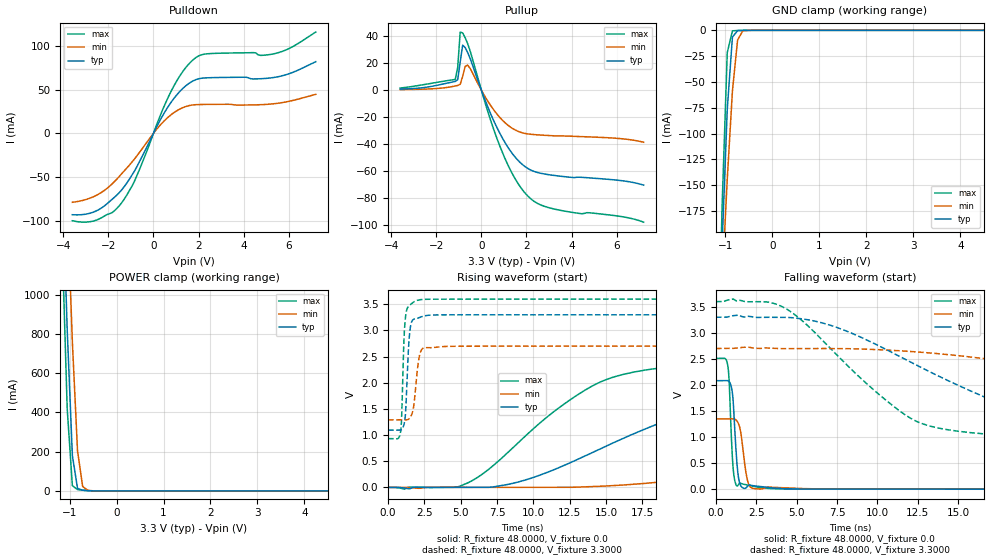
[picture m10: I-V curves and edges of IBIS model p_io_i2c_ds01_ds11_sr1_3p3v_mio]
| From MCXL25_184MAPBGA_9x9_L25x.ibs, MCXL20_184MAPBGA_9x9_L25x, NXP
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[Model] p_io_i2c_ds01_ds11_sr1_3p3v_mio
|   Model p_io_i2c_ds01_ds11_sr1_3p3v_mio
| This model was characterised for following simulation conditions:
| External (pad) voltage:
|   - Typ: 3.3V,   - Min: 2.7V,   - Max: 3.6V
| Library cells for typ/min/max conditions are connected as defined below:
|  pad - External Pad
|  ipp_do_lv - Core Input
|  ipp_obe_lv - Output Buffer Enable
|  IOGC - NC
|  REFH3V3 - REFH3V3
|  REFL3V3 - REFL3V3
|  ZI - NC
|  abut_ncal_vddio[1] - vddio
|  abut_ncal_vddio[2] - vddio
|  abut_ncal_vddio[3] - vssio
|  abut_ncal_vddio[4] - vddio
|  abut_ncal_vddio[5] - vddio
|  abut_ncal_vddio[6] - vssio
|  abut_pcal_vddio[1] - vssio
|  abut_pcal_vddio[2] - vssio
|  abut_pcal_vddio[3] - vddio
|  abut_pcal_vddio[4] - vssio
|  abut_pcal_vddio[5] - vssio
|  abut_pcal_vddio[6] - vddio
|  ipp_do_1p8v - ipp_do_1p8v
|  ipp_dse_lv[0] - vdd_lv
|  ipp_dse_lv[1] - vdd_lv
|  ipp_eftd_lv - NC
|  ipp_ina_mux_vddio - NC
|  ipp_ina_mux_vddio[0] - NC
|  ipp_ina_mux_vddio[1] - NC
|  ipp_ina_r0_vddio - NC
|  ipp_ina_r0a_vddio - NC
|  ipp_ina_r0b_vddio - NC
|  ipp_ina_r0c_vddio - NC
|  ipp_ina_r0d_vddio - NC
|  ipp_ina_r0e_vddio - NC
|  ipp_ina_r0f_vddio - NC
|  ipp_ina_r300_vddio - NC
|  ipp_ina_r300a_vddio - NC
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Model_type I/O
Polarity   Non-Inverting
Enable   Active-High
Vinl =   0.9900V
Vinh =   2.3100V
Vmeas =  1.6500V
Cref =   30.0000pF
Rref =   1.0000M
Vref =   3.3000V
C_comp   1.4149pF   1.3702pF   1.4746pF
|C_comp_pullup   0.5855pF   0.6309pF   0.5569pF
|C_comp_pulldown   0.7315pF   0.7413pF   0.7170pF
[Model Spec]
| variable   typ   min   max
Vinh   2.3100V   1.8900V   2.5200V
Vinl   0.9900V   0.8100V   1.0800V
[Temperature Range]   25.0000   0.1250k   -40.0000
[Voltage Range]   3.3000V   2.7000V   3.6000V
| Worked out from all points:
|   slope of the pulldown table from 0 to 0.495 V, typ, clamps not added: 20.5 ohm
|   slope of the pullup table from 0 to 0.495 V, typ, clamps not added: 23.9 ohm
|   GND clamp passes 1 mA (typ) near -0.75 V on its own axis
|   POWER clamp passes 1 mA (typ) near -0.57 V on its own axis
|   rising waveform, R_fixture 48.0000, V_fixture 0.0: 20-80 % time 11.6ns typ, 24.8ns min, 6.96ns max; typ from 0 V to 2.08 V
|   rising waveform, R_fixture 48.0000, V_fixture 3.3000: 20-80 % time 229ps typ, 322ps min, 191ps max; typ from 1.09 V to 3.3 V
|   falling waveform, R_fixture 48.0000, V_fixture 0.0: 20-80 % time 251ps typ, 343ps min, 212ps max; typ from 2.08 V to 0 V
|   falling waveform, R_fixture 48.0000, V_fixture 3.3000: 20-80 % time 9.25ns typ, 20.1ns min, 5.61ns max; typ from 3.3 V to 1.09 V
[Pulldown]
|Voltage   I(typ)   I(min)   I(max)
-3.6V     -93.31mA   -79.05mA   -100.2mA
-2.5V     -88.48mA   -70.63mA   -99.19mA
-1.84V    -75.78mA   -58.1mA    -91mA
-1.4V     -64.51mA   -45.95mA   -79.27mA
-850mV    -43.59mA   -29.61mA   -55.29mA
140mV     7.403mA    4.641mA    9.826mA
800mV     36.32mA    21.74mA    49.15mA
1.35V     52.7mA     30.01mA    72.7mA
1.79V     60.61mA    32.73mA    85.13mA
2.45V     63.81mA    33.25mA    91.42mA
5.42V     64.46mA    34.22mA    91.77mA
7.2V      82.23mA    44.78mA    116.2mA
[Pullup]
|Voltage   I(typ)   I(min)   I(max)
-3.6V     785.4uA    423.2uA    1.608mA
-1.16V    6.455mA    3.098mA    7.926mA
-1.05V    7.777mA    3.482mA    16.99mA
-940mV    20.9mA     4.372mA    43.05mA
-830mV    33.33mA    10.25mA    42.41mA
-720mV    31.61mA    17.65mA    38.91mA
-610mV    27.98mA    18.58mA    34.56mA
820mV     -32.01mA   -20.24mA   -41.48mA
1.48V     -49.28mA   -29.34mA   -65.19mA
2.03V     -57.72mA   -32.35mA   -77.98mA
3.24V     -63.24mA   -33.85mA   -88.14mA
7.2V      -70.41mA   -38.61mA   -97.87mA
[GND_clamp]
|Voltage   I(typ)   I(min)   I(max)
-3.6V     -4.327A    -3.181A    -5.901A
-1.18V    -358.9mA   -350.6mA   -379.3mA
-1.07V    -208.2mA   -244.2mA   -170.8mA
-960mV    -76.59mA   -144.3mA   -21.58mA
-850mV    -6.561mA   -58.74mA   -511.4uA
-740mV    -273.3uA   -9.382mA   -185.3uA
-630mV    -73.8uA    -593.1uA   -77.52uA
-410mV    -3.432uA   -9.016uA   -2.104uA
7.2V      0A         0A         0A
[POWER_clamp]
|Voltage   I(typ)   I(min)   I(max)
-3.6V     20.44A     18.76A     22.48A
-1.16V    1.647A     2.216A     1.289A
-1.05V    823.6mA    1.482A     419.2mA
-940mV    180.4mA    758.9mA    26.72mA
-830mV    12.56mA    202.9mA    6.794mA
-720mV    3.422mA    22.23mA    3.58mA
-610mV    1.373mA    2.923mA    1.344mA
7.2V      0A         0A         0A
[Ramp]
| variable   typ   min   max
dV/dt_r  1.2488/11.6455n   0.8046/24.8064n   1.5056/6.9631n
dV/dt_f  1.3236/9.2490n   0.8437/20.0953n   1.6008/5.6139n
R_load = 48.0000
[Rising Waveform]
R_fixture= 48.0000
V_fixture= 0.0
V_fixture_min= 0.0
V_fixture_max= 0.0
|time   V(typ)   V(min)   V(max)
0s        1.113nV    81.31nV    3.704nV
4.822ns   -93.59uV   -374.1uV   11.23mV
8.815ns   92.04mV    -10.93uV   815.9mV
11.69ns   369.3mV    447.9uV    1.507V
14.6ns    735.1mV    20.79mV    2.013V
21.96ns   1.546V     199.7mV    2.365V
32.5ns    1.913V     598.4mV    2.465V
43.62ns   2.011V     972.6mV    2.494V
54.48ns   2.049V     1.147V     2.504V
135.1ns   2.081V     1.341V     2.509V
[Rising Waveform]
R_fixture= 48.0000
V_fixture= 3.3000
V_fixture_min= 2.7000
V_fixture_max= 3.6000
|time   V(typ)   V(min)   V(max)
0s        1.094V     1.29V      932mV
866.7ps   1.095V     1.29V      1.071V
939.6ps   1.107V     1.29V      1.384V
1.102ns   1.21V      1.29V      2.874V
1.277ns   1.85V      1.29V      3.385V
1.419ns   2.721V     1.304V     3.464V
1.57ns    3.114V     1.359V     3.502V
2.123ns   3.243V     2.462V     3.584V
2.381ns   3.269V     2.655V     3.593V
135.1ns   3.3V       2.7V       3.6V
[Falling Waveform]
R_fixture= 48.0000
V_fixture= 0.0
V_fixture_min= 0.0
V_fixture_max= 0.0
|time   V(typ)   V(min)   V(max)
0s        2.082V     1.348V     2.509V
733.5ps   2.082V     1.348V     2.368V
812.6ps   2.066V     1.348V     2.09V
1.018ns   1.843V     1.35V      597.4mV
1.237ns   760.7mV    1.329V     88.39mV
1.354ns   314mV      1.282V     68.91mV
1.486ns   100.6mV    1.167V     119.5mV
2.057ns   79.63mV    72.47mV    73.68mV
3.334ns   29.04mV    40.43mV    12.65mV
135.1ns   124.7nV    2.869uV    13.74nV
[Falling Waveform]
R_fixture= 48.0000
V_fixture= 3.3000
V_fixture_min= 2.7000
V_fixture_max= 3.6000
|time   V(typ)   V(min)   V(max)
0s        3.3V       2.7V       3.6V
3.896ns   3.299V     2.698V     3.531V
7.01ns    3.154V     2.699V     2.727V
12.22ns   2.412V     2.639V     1.332V
17.62ns   1.645V     2.466V     1.039V
20.46ns   1.405V     2.342V     998.1mV
25.67ns   1.251V     2.093V     962.8mV
36.08ns   1.151V     1.644V     940.7mV
46.79ns   1.118V     1.462V     934.8mV
135.1ns   1.094V     1.294V     932mV
